(* Logix 5000 AddOnInstructionDefinition export Banner_K50Display_Param_v4; software revision 33.03 *)

TYPE Banner_IOL_Port_v4 :   // UDT that has all of the data items necessary to communicate with a specific Port on a IO-Link Master
STRUCT
   Port_Controlled : INT;   // Each bit represents a port on an IO-Link Master. Set to 1 to tell AOI to control that port.
   Port_Activate : INT;   // Each bit represents a port on an IO-Link Master. When ON that port will process any commands in queue.
   Port_Read : INT;   // Each bit represents a port on an IO-Link Master. Used to determine when device AOI has requested a Read command.
   Port_Write : INT;   // Each bit represents a port on an IO-Link Master. Used to determine when device AOI has requested a Write command.
   Port_RW_Complete : INT;   // Each bit represents a port on an IO-Link Master. Tells device AOI that Read or Write request has been completed.
   Port_Device_Read : INT;
   Data_Transfer : SINT[190];   // Array to transfer data from IO-Master to device AOIs.
END_STRUCT
END_TYPE

TYPE Banner_K50Display_Display_v4 :   // UDT that covers Display Configuration parameters.
STRUCT
   Intensity : SINT;   // 0 = Low, 1 = Medium, 2 = High, 3 = Ultra High
   Orientation : SINT;   // 0 = Standard, 1 = Flipped
   Scroll_Speed : SINT;   // 0 = Off, 1 = Slow, 2 = Medium, 3 = Fast
   Startup_Message : SINT;   // 0 = Off, 1 = Comms Parameter, 2 = Custom
   Startup_String_Delay : DINT;   // 0 to 65535 ms
   Encoding : SINT;   // 0 = ASCII, 1 = Numeric
   Decimal_Type_1 : SINT;   // 0 = Off, 1 = On, 2 = Flash, 3 = Communication, 4 = Power + Communication.
   Decimal_Type_2 : SINT;   // 0 = Off, 1 = On, 2 = Flash, 3 = Communication, 4 = Power + Communication.
   Decimal_Type_3 : SINT;   // 0 = Off, 1 = On, 2 = Flash, 3 = Communication, 4 = Power + Communication.
   Decimal_Type_4 : SINT;   // 0 = Off, 1 = On, 2 = Flash, 3 = Communication, 4 = Power + Communication.
   Startup_String : STRING;
END_STRUCT
END_TYPE

TYPE Banner_K50Display_RD_v4 :   // UDT with all of the Read only parameters for K50 Pro Display.
STRUCT
   Master_Cycle_Time : INT;
   Min_Cycle_Time : INT;
   M_Sequence_Capability : INT;
   IO_Link_Version_ID : INT;
   Process_Data_Input_Length : INT;
   Process_Data_Output_Length : INT;
   Combined_Vendor_ID : DINT;   // IO-Link Vendor ID
   Vendor_ID1 : INT;
   Vendor_ID2 : INT;
   Combined_Device_ID : DINT;   // IO-Link Device ID
   Device_ID1 : INT;
   Device_ID2 : INT;
   Device_ID3 : INT;
   Serial_Number : STRING;
END_STRUCT
END_TYPE

TYPE Banner_K50Display_SP_v4 :   // UDT for K50 Pro Display with the State Parameters structure.
STRUCT
   Type : SINT;   // 0 = Off, 1 = Steady, 2 = Flash, 3 = Two Color Flash, 4 = 50/50, 5 = 50/50 Rotate, 6 = Chase, 7 = Intensity Sweep, 8 = Color Sweep, 9 = Sequence, 10 = Wave, 11 = Double Wave, 12 = Steady Area 1, 13 = Steady Area 2, 14 Alternate Area 1 Area 2
   Direction : SINT;   // 0 = CCW, 1 = CW.
   Pattern : SINT;   // 0 = Flash, 1 = Strobe, 2 = Three Pulse, 3 = SOS, 4 = Random.
   Speed : SINT;   // 0 = Slow, 1 = Medium, 2 = Fast, 3 = Custom.
   Off_Delay_Type : SINT;   // 0 =Leading Edge, 1 = Trailing Edge.
   Off_Delay : DINT;   // 0 to 65535 in ms. Length of time before the device returns to 'touch inactive' state after button is released.
   Static_Sequence : INT;   // 0 to 255. Value describing the LED position of the device.
   Sequence_Start_Location : SINT;   // 0 = LED1, 1 = LED2, 2 = LED3, 3 = LED4, 4 = LED5, 5 = LED6, 6 = LED7, 7 = LED8.
   Color_1 : SINT;   // 0 = Green, 1 = Red, 2 = Orange, 3 = Amber, 4 = Yellow, 5 = Lime Green, 6 = Spring Green, 7 = Cyan, 8 = SKy Blue, 9 = Blue, 10 = Violet, 11 = Magenta, 12 = Rose, 13 = White, 14 Custom 1, 15 = Custom 2.
   Color_1_Intensity : SINT;   // 0 = High, 1 = Medium, 2 = Low, 3 = Off, 4 = Custom.
   Color_2 : SINT;   // 0 = Green, 1 = Red, 2 = Orange, 3 = Amber, 4 = Yellow, 5 = Lime Green, 6 = Spring Green, 7 = Cyan, 8 = SKy Blue, 9 = Blue, 10 = Violet, 11 = Magenta, 12 = Rose, 13 = White, 14 Custom 1, 15 = Custom 2.
   Color_2_Intensity : SINT;   // 0 = High, 1 = Medium, 2 = Low, 3 = Off, 4 = Custom.
END_STRUCT
END_TYPE

TYPE Banner_K50Display_v4 :   // UDT with all of the parameters for K50 Pro Display.
STRUCT
   Initial_Global_Read : BOOL;   // Determines if all of the IO-Link data has been read into the PLC yet
   Command : INT;   // Value placed in here will activate a read or write to a specifc IO-Link Index
   Read : Banner_K50Display_RD_v4;   // All read data
   Write : Banner_K50Display_WD_v4;   // All data that can be written to.
   Archive : Banner_K50Display_WD_v4;   // Archive of the write data.
   Reset : BOOL;
END_STRUCT
END_TYPE

TYPE Banner_K50Display_WD_v4 :   // UDT that stores the Write Data for a K50 Pro Display.
STRUCT
   System_Command : INT;   // See IODD file for list of commands that can be activated via the System Command interface
   Parameter_Access_Lock : SINT;   // Write access to all read/write parameters is block when this bit is ON.
   Data_Storage_Lock : SINT;   // Data storage mechanism is inhibited when bit is ON.
   Local_Parameterization_Lock : SINT;   // Parameteriation via local control elementes is inhibited.
   Local_User_Interface_Lock : SINT;   // Operation of the hmi on the device is disabled.
   Operation_Mode : SINT;   // 0 = Multicolor, 1 = Four State Full Logic, 2 = Advanced, 3 = LED Control, 4 = Demo.
   Custom_Intensity : SINT;   // 0 to 100 %
   Custom_Flash_Rate : INT;   // Range 5 to 200 (.5 to 20 converted rate).
   Restrict_to_Gamut : SINT;   // 0 = Off, 1 = On.
   Touch_Sensitivity : SINT;   // 0 = Low, 1 = Standard, 2 = High.
   Function_1 : SINT;   // 0 = Momentary, 1 = Latched.
   Mute_Enable_1 : SINT;   // 0 = Off, 1 = On.
   Function_2 : SINT;   // 0 = Momentary, 1 = Latched.
   Mute_Enable_2 : SINT;   // 0 = Off, 1 = On.
   On_Delay_1 : DINT;   // 0 to 65535 in ms. Length of time the touch button needs to be pressed to trigger touch active state.
   On_Delay_2 : DINT;   // 0 to 65535 in ms. Length of time the touch button needs to be pressed to trigger touch active state.
   Output_State : SINT;   // 0 = NC, 1 = NO
   Off_Delay_Type_1 : SINT;   // 0 - Leading Edge, 1 = Trailing Edge
   Off_Delay_Type_2 : SINT;   // 0 - Leading Edge, 1 = Trailing Edge
   Off_Delay_1 : DINT;   // Length of time before device returns to touch inactive
   Off_Delay_2 : DINT;   // Length of time before device returns to touch inactive
   State_Parameters : Banner_K50Display_SP_v4[6];   // State Parameters. 1 through 4 will have values.
   CC1_Red : INT;   // 0-255. Custom 1 Red.
   CC1_Green : INT;   // 0-255. Custom 1 Green.
   CC1_Blue : INT;   // 0-255. Custom 1 Blue.
   CC2_Red : INT;   // 0-255. Custom 2 Red.
   CC2_Green : INT;   // 0-255. Custom 2 Green.
   CC2_Blue : INT;   // 0-255. Custom 2 Blue.
   Display_Config : Banner_K50Display_Display_v4;
END_STRUCT
END_TYPE

ADD_ON_INSTRUCTION Banner_K50Display_Param_v4   (* revision 4.2, vendor Banner Engineering *)
// AOI to read and write parameter data to an IO-Link K50 Pro Display.
// Revision note:
// Resolved transfer array index issue.
VAR_IN_OUT
   K50 : Banner_K50Display_v4; {required}
   Port_Data : Banner_IOL_Port_v4; {required}
END_VAR
VAR_INPUT
   Port : DINT; {required}
END_VAR
VAR
   Local_Control : DINT; {access None}
   Global_Read_Command_Value : INT; {access None}
   Global_Write_Command_Value : INT; {access None}
   Command_Being_Processed : BOOL; {access None}
   Update_Archive : BOOL; {access None}
   Index_Write_Control : DINT; {access None}
   Index_Write_Inprocess : INT; {access None}
   Temp_Excess_Gain : DINT[2]; {access None}
   Inprocess_Index : DINT; {access None}
   SP_Index : DINT; {access None}   // State Parameters Index
   SP_Write_Index : DINT; {access None}
   SP_R_Index : DINT; {access None}
   SP_W_Index : DINT; {access None}
END_VAR

ROUTINE Logic   (* ladder *)
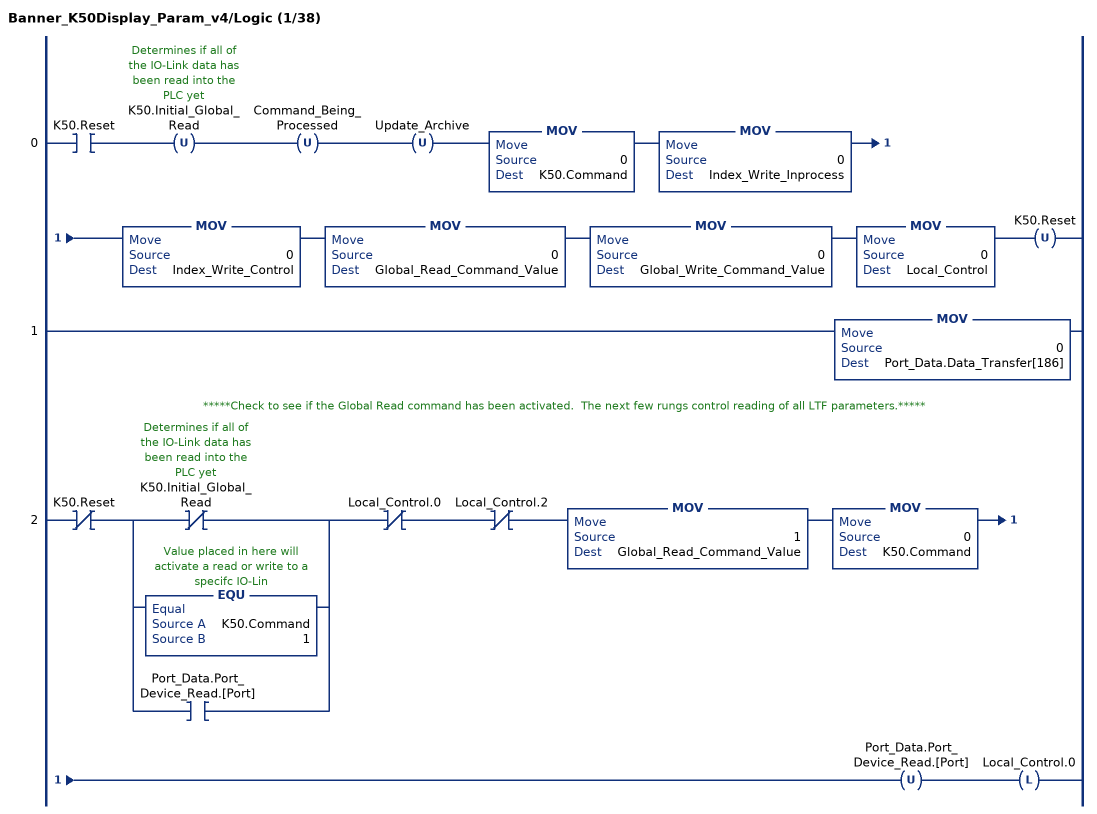
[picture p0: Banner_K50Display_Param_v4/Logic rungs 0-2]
   0: XIC(K50.Reset)OTU(K50.Initial_Global_Read)OTU(Command_Being_Processed)OTU(Update_Archive)MOV(0,K50.Command)MOV(0,Index_Write_Inprocess)MOV(0,Index_Write_Control)MOV(0,Global_Read_Command_Value)MOV(0,Global_Write_Command_Value)MOV(0,Local_Control)OTU(K50.Reset);
   1: MOV(0,Port_Data.Data_Transfer[186]);
   // *****Check to see if the Global Read command has been activated.  The next few rungs control reading of all LTF parameters.*****
   2: XIO(K50.Reset)[XIO(K50.Initial_Global_Read) ,EQU(K50.Command,1) ,XIC(Port_Data.Port_Device_Read.[Port]) ]XIO(Local_Control.0)XIO(Local_Control.2)MOV(1,Global_Read_Command_Value)MOV(0,K50.Command)OTU(Port_Data.Port_Device_Read.[Port])OTL(Local_Control.0);
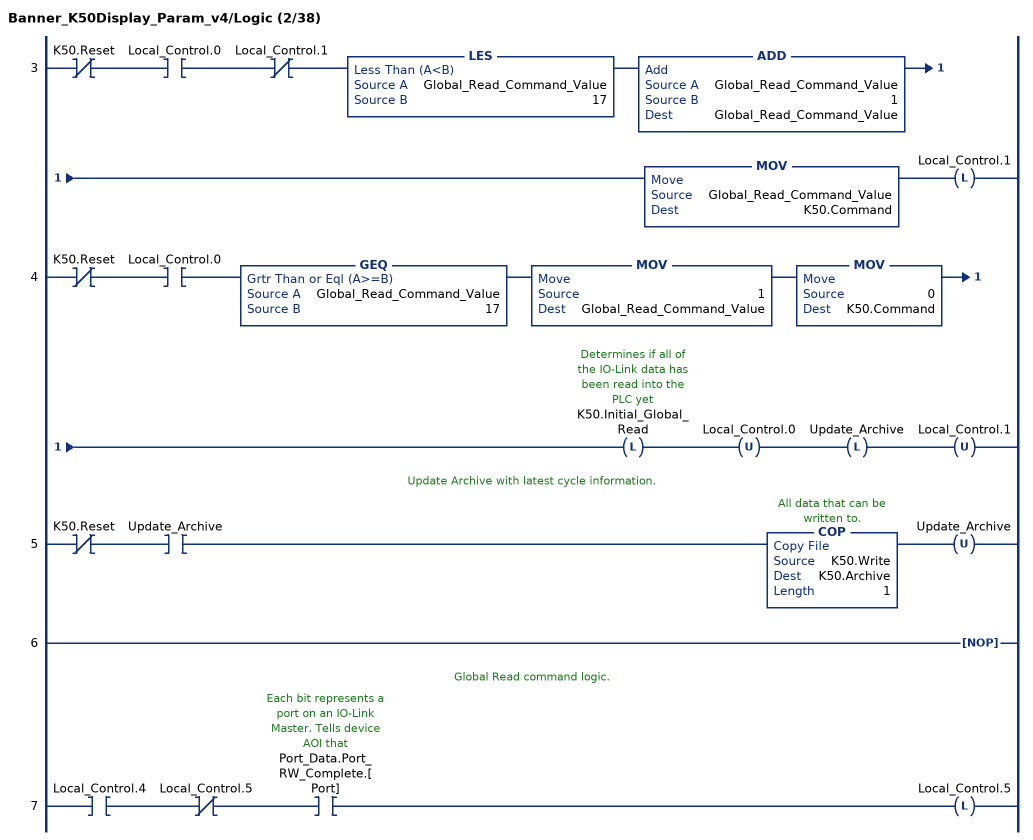
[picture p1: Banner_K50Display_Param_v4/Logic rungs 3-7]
   3: XIO(K50.Reset)XIC(Local_Control.0)XIO(Local_Control.1)LES(Global_Read_Command_Value,17)ADD(Global_Read_Command_Value,1,Global_Read_Command_Value)MOV(Global_Read_Command_Value,K50.Command)OTL(Local_Control.1);
   4: XIO(K50.Reset)XIC(Local_Control.0)GEQ(Global_Read_Command_Value,17)MOV(1,Global_Read_Command_Value)MOV(0,K50.Command)OTL(K50.Initial_Global_Read)OTU(Local_Control.0)OTL(Update_Archive)OTU(Local_Control.1);
   // Update Archive with latest cycle information.
   5: XIO(K50.Reset)XIC(Update_Archive)COP(K50.Write,K50.Archive,1)OTU(Update_Archive);
   6: NOP();
   // Global Read command logic.
   7: XIC(Local_Control.4)XIO(Local_Control.5)XIC(Port_Data.Port_RW_Complete.[Port])OTL(Local_Control.5);
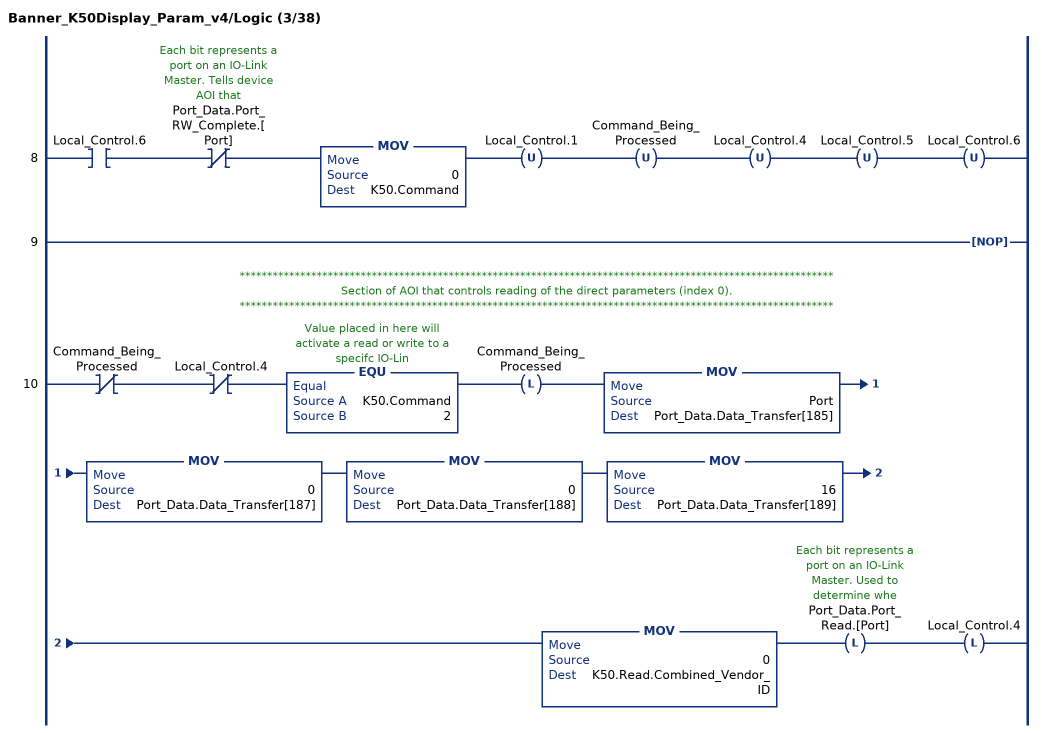
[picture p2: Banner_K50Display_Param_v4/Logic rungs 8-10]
   8: XIC(Local_Control.6)XIO(Port_Data.Port_RW_Complete.[Port])MOV(0,K50.Command)OTU(Local_Control.1)OTU(Command_Being_Processed)OTU(Local_Control.4)OTU(Local_Control.5)OTU(Local_Control.6);
   9: NOP();
   // ************************************************************************************************************
   // Section of AOI that controls reading of the direct parameters (index 0).
   // ************************************************************************************************************
   10: XIO(Command_Being_Processed)XIO(Local_Control.4)EQU(K50.Command,2)OTL(Command_Being_Processed)MOV(Port,Port_Data.Data_Transfer[185])MOV(0,Port_Data.Data_Transfer[187])MOV(0,Port_Data.Data_Transfer[188])MOV(16,Port_Data.Data_Transfer[189])MOV(0,K50.Read.Combined_Vendor_ID)OTL(Port_Data.Port_Read.[Port])OTL(Local_Control.4);
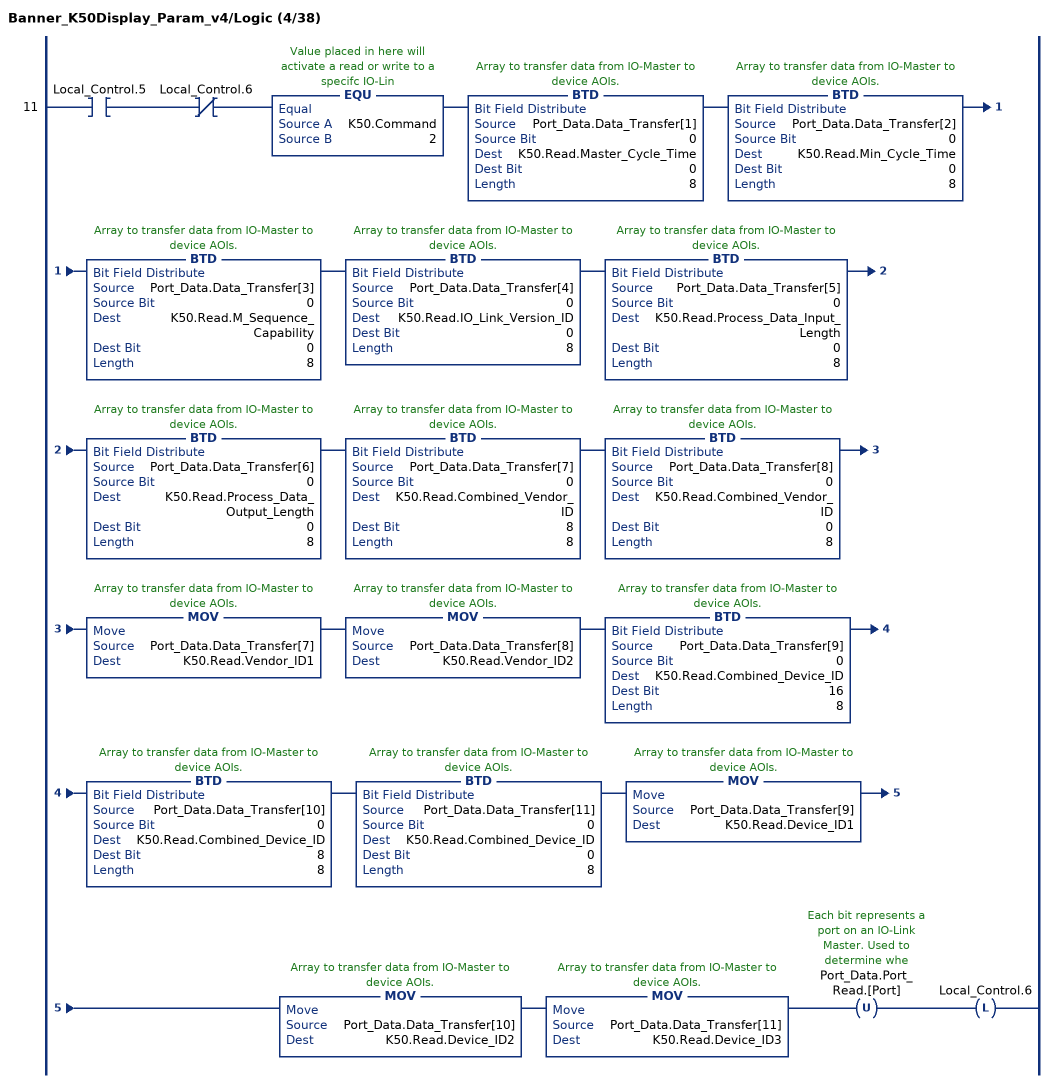
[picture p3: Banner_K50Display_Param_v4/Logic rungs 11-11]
   11: XIC(Local_Control.5)XIO(Local_Control.6)EQU(K50.Command,2)BTD(Port_Data.Data_Transfer[1],0,K50.Read.Master_Cycle_Time,0,8)BTD(Port_Data.Data_Transfer[2],0,K50.Read.Min_Cycle_Time,0,8)BTD(Port_Data.Data_Transfer[3],0,K50.Read.M_Sequence_Capability,0,8)BTD(Port_Data.Data_Transfer[4],0,K50.Read.IO_Link_Version_ID,0,8)BTD(Port_Data.Data_Transfer[5],0,K50.Read.Process_Data_Input_Length,0,8)BTD(Port_Data.Data_Transfer[6],0,K50.Read.Process_Data_Output_Length,0,8)BTD(Port_Data.Data_Transfer[7],0,K50.Read.Combined_Vendor_ID,8,8)BTD(Port_Data.Data_Transfer[8],0,K50.Read.Combined_Vendor_ID,0,8)MOV(Port_Data.Data_Transfer[7],K50.Read.Vendor_ID1)MOV(Port_Data.Data_Transfer[8],K50.Read.Vendor_ID2)BTD(Port_Data.Data_Transfer[9],0,K50.Read.Combined_Device_ID,16,8)BTD(Port_Data.Data_Transfer[10],0,K50.Read.Combined_Device_ID,8,8)BTD(Port_Data.Data_Transfer[11],0,K50.Read.Combined_Device_ID,0,8)MOV(Port_Data.Data_Transfer[9],K50.Read.Device_ID1)MOV(Port_Data.Data_Transfer[10],K50.Read.Device_ID2)MOV(Port_Data.Data_Transfer[11],K50.Read.Device_ID3)OTU(Port_Data.Port_Read.[Port])OTL(Local_Control.6);
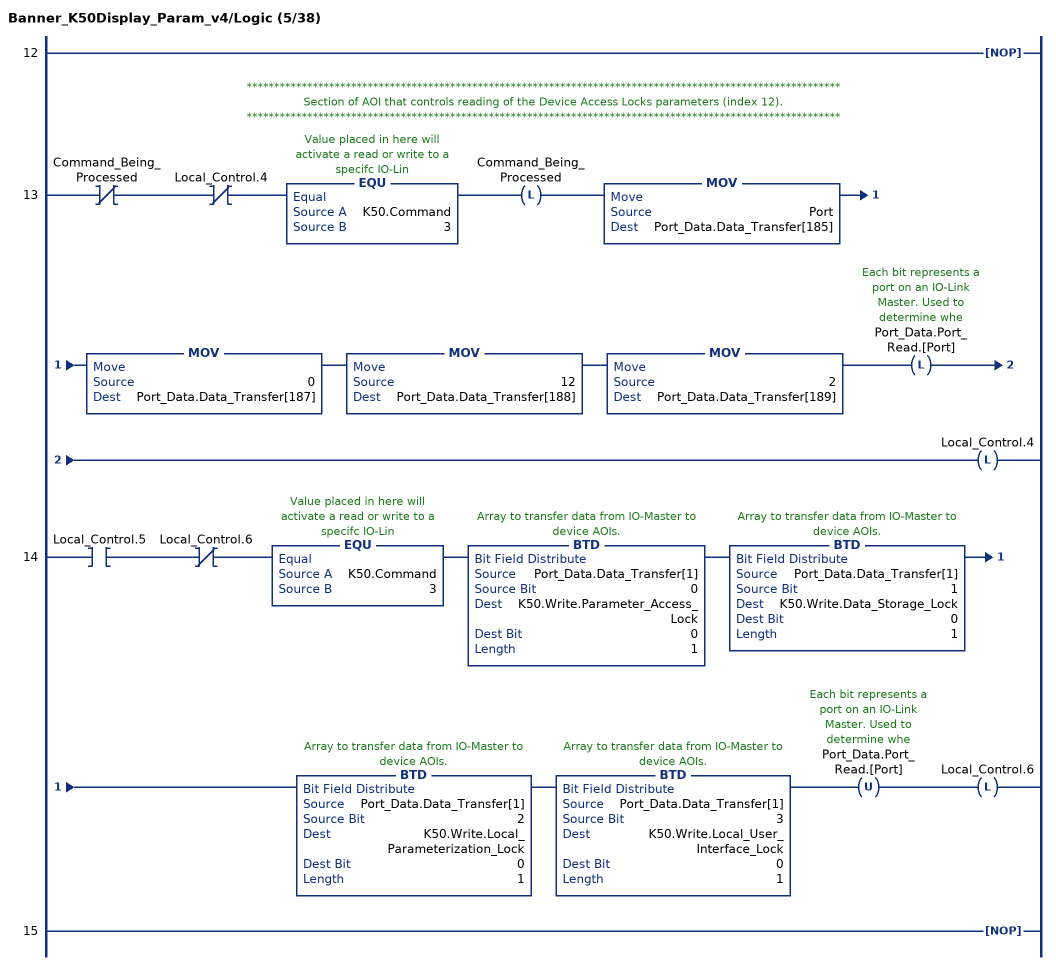
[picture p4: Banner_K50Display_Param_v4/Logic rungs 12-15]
   12: NOP();
   // ************************************************************************************************************
   // Section of AOI that controls reading of the Device Access Locks parameters (index 12).
   // ************************************************************************************************************
   13: XIO(Command_Being_Processed)XIO(Local_Control.4)EQU(K50.Command,3)OTL(Command_Being_Processed)MOV(Port,Port_Data.Data_Transfer[185])MOV(0,Port_Data.Data_Transfer[187])MOV(12,Port_Data.Data_Transfer[188])MOV(2,Port_Data.Data_Transfer[189])OTL(Port_Data.Port_Read.[Port])OTL(Local_Control.4);
   14: XIC(Local_Control.5)XIO(Local_Control.6)EQU(K50.Command,3)BTD(Port_Data.Data_Transfer[1],0,K50.Write.Parameter_Access_Lock,0,1)BTD(Port_Data.Data_Transfer[1],1,K50.Write.Data_Storage_Lock,0,1)BTD(Port_Data.Data_Transfer[1],2,K50.Write.Local_Parameterization_Lock,0,1)BTD(Port_Data.Data_Transfer[1],3,K50.Write.Local_User_Interface_Lock,0,1)OTU(Port_Data.Port_Read.[Port])OTL(Local_Control.6);
   15: NOP();
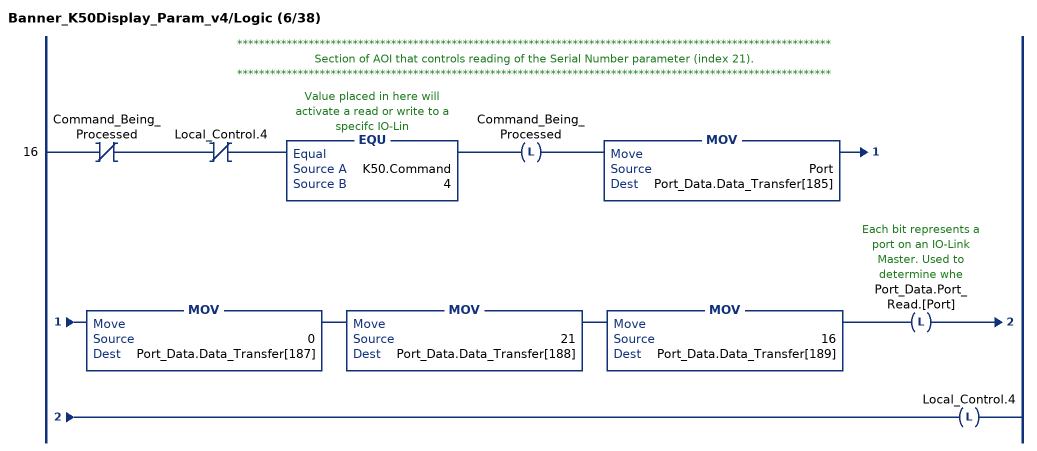
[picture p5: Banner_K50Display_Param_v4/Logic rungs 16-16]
   // ************************************************************************************************************
   // Section of AOI that controls reading of the Serial Number parameter (index 21).
   // ************************************************************************************************************
   16: XIO(Command_Being_Processed)XIO(Local_Control.4)EQU(K50.Command,4)OTL(Command_Being_Processed)MOV(Port,Port_Data.Data_Transfer[185])MOV(0,Port_Data.Data_Transfer[187])MOV(21,Port_Data.Data_Transfer[188])MOV(16,Port_Data.Data_Transfer[189])OTL(Port_Data.Port_Read.[Port])OTL(Local_Control.4);
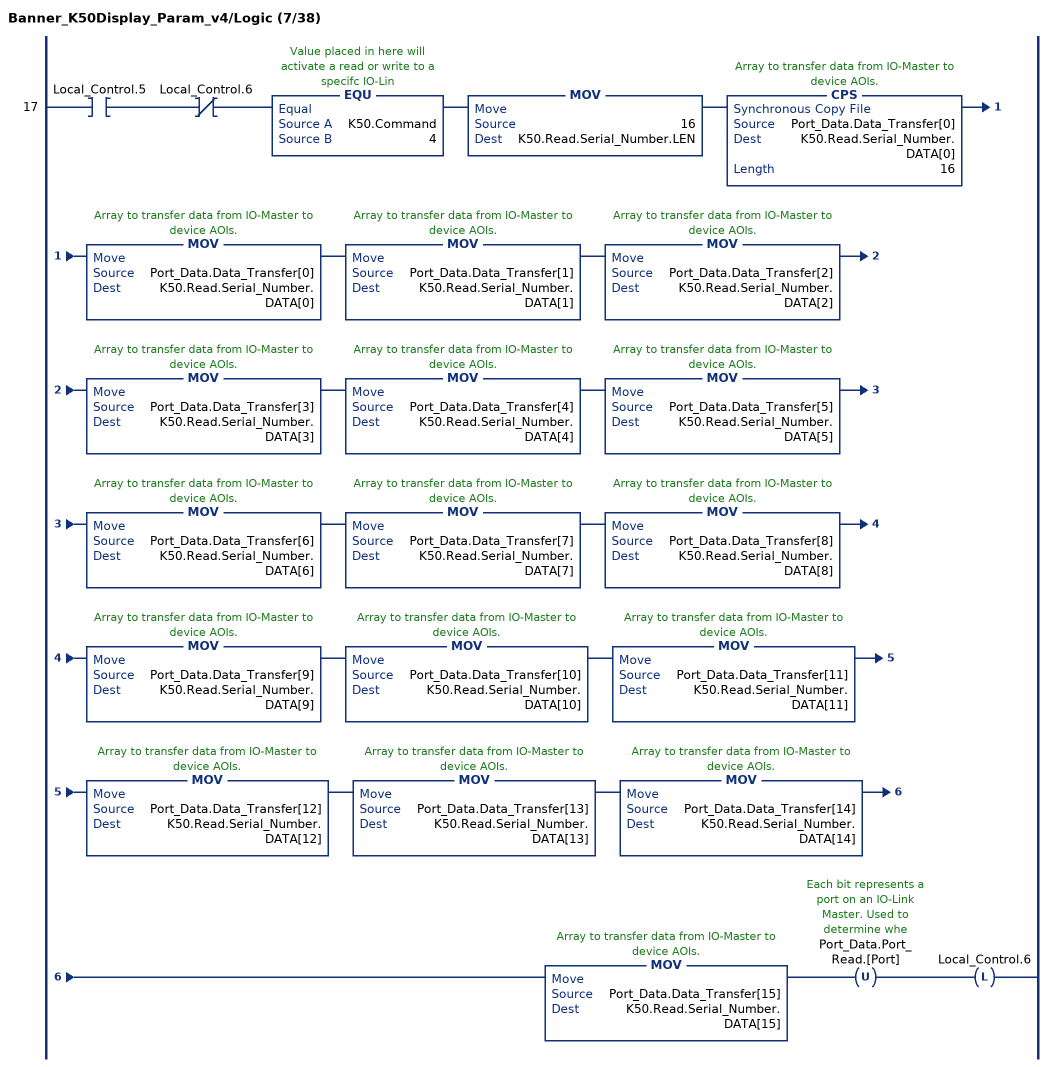
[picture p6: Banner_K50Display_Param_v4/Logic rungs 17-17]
   17: XIC(Local_Control.5)XIO(Local_Control.6)EQU(K50.Command,4)MOV(16,K50.Read.Serial_Number.LEN)CPS(Port_Data.Data_Transfer[0],K50.Read.Serial_Number.DATA[0],16)MOV(Port_Data.Data_Transfer[0],K50.Read.Serial_Number.DATA[0])MOV(Port_Data.Data_Transfer[1],K50.Read.Serial_Number.DATA[1])MOV(Port_Data.Data_Transfer[2],K50.Read.Serial_Number.DATA[2])MOV(Port_Data.Data_Transfer[3],K50.Read.Serial_Number.DATA[3])MOV(Port_Data.Data_Transfer[4],K50.Read.Serial_Number.DATA[4])MOV(Port_Data.Data_Transfer[5],K50.Read.Serial_Number.DATA[5])MOV(Port_Data.Data_Transfer[6],K50.Read.Serial_Number.DATA[6])MOV(Port_Data.Data_Transfer[7],K50.Read.Serial_Number.DATA[7])MOV(Port_Data.Data_Transfer[8],K50.Read.Serial_Number.DATA[8])MOV(Port_Data.Data_Transfer[9],K50.Read.Serial_Number.DATA[9])MOV(Port_Data.Data_Transfer[10],K50.Read.Serial_Number.DATA[10])MOV(Port_Data.Data_Transfer[11],K50.Read.Serial_Number.DATA[11])MOV(Port_Data.Data_Transfer[12],K50.Read.Serial_Number.DATA[12])MOV(Port_Data.Data_Transfer[13],K50.Read.Serial_Number.DATA[13])MOV(Port_Data.Data_Transfer[14],K50.Read.Serial_Number.DATA[14])MOV(Port_Data.Data_Transfer[15],K50.Read.Serial_Number.DATA[15])OTU(Port_Data.Port_Read.[Port])OTL(Local_Control.6);
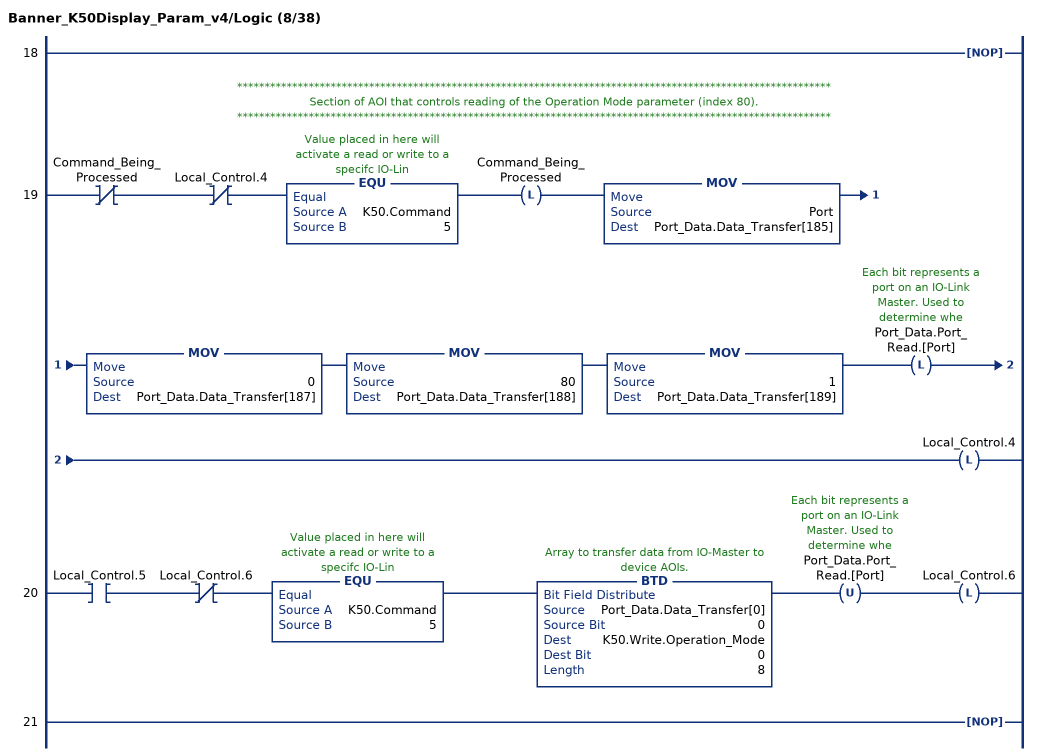
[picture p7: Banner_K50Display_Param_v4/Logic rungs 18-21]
   18: NOP();
   // ************************************************************************************************************
   // Section of AOI that controls reading of the Operation Mode parameter (index 80).
   // ************************************************************************************************************
   19: XIO(Command_Being_Processed)XIO(Local_Control.4)EQU(K50.Command,5)OTL(Command_Being_Processed)MOV(Port,Port_Data.Data_Transfer[185])MOV(0,Port_Data.Data_Transfer[187])MOV(80,Port_Data.Data_Transfer[188])MOV(1,Port_Data.Data_Transfer[189])OTL(Port_Data.Port_Read.[Port])OTL(Local_Control.4);
   20: XIC(Local_Control.5)XIO(Local_Control.6)EQU(K50.Command,5)BTD(Port_Data.Data_Transfer[0],0,K50.Write.Operation_Mode,0,8)OTU(Port_Data.Port_Read.[Port])OTL(Local_Control.6);
   21: NOP();
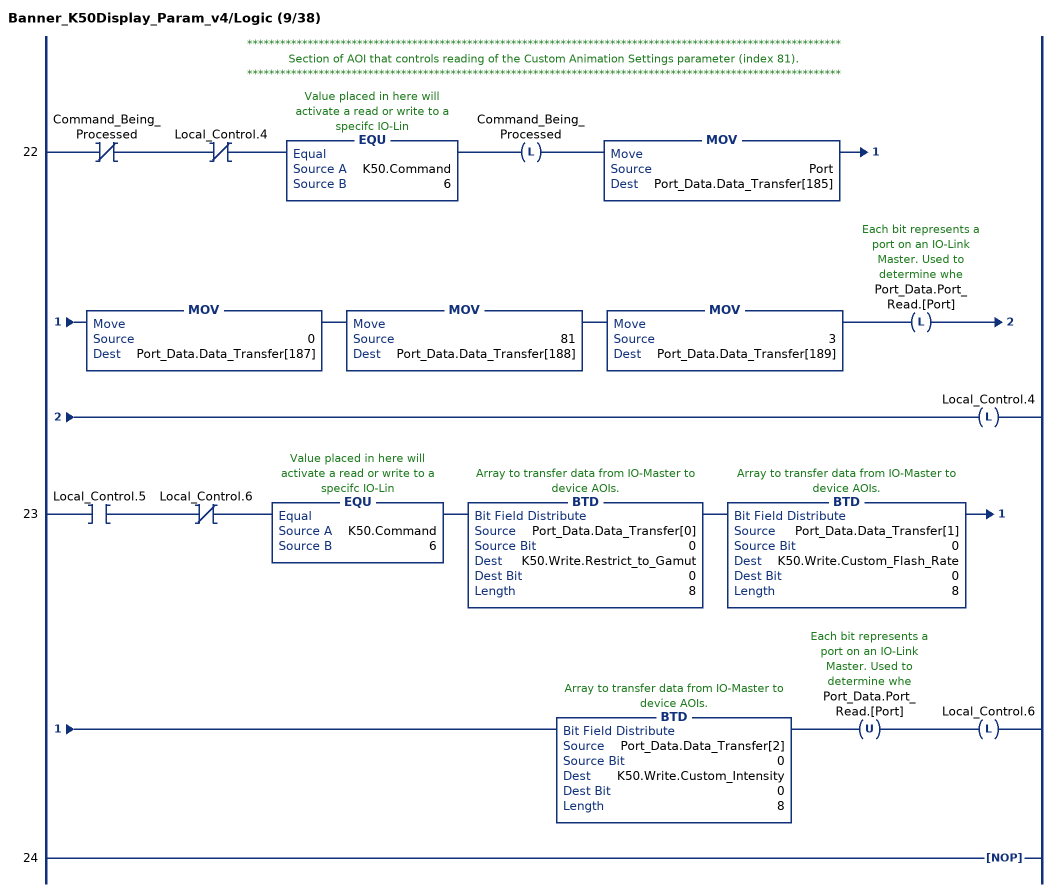
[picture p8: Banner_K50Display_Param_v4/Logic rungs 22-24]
   // ************************************************************************************************************
   // Section of AOI that controls reading of the Custom Animation Settings parameter (index 81).
   // ************************************************************************************************************
   22: XIO(Command_Being_Processed)XIO(Local_Control.4)EQU(K50.Command,6)OTL(Command_Being_Processed)MOV(Port,Port_Data.Data_Transfer[185])MOV(0,Port_Data.Data_Transfer[187])MOV(81,Port_Data.Data_Transfer[188])MOV(3,Port_Data.Data_Transfer[189])OTL(Port_Data.Port_Read.[Port])OTL(Local_Control.4);
   23: XIC(Local_Control.5)XIO(Local_Control.6)EQU(K50.Command,6)BTD(Port_Data.Data_Transfer[0],0,K50.Write.Restrict_to_Gamut,0,8)BTD(Port_Data.Data_Transfer[1],0,K50.Write.Custom_Flash_Rate,0,8)BTD(Port_Data.Data_Transfer[2],0,K50.Write.Custom_Intensity,0,8)OTU(Port_Data.Port_Read.[Port])OTL(Local_Control.6);
   24: NOP();
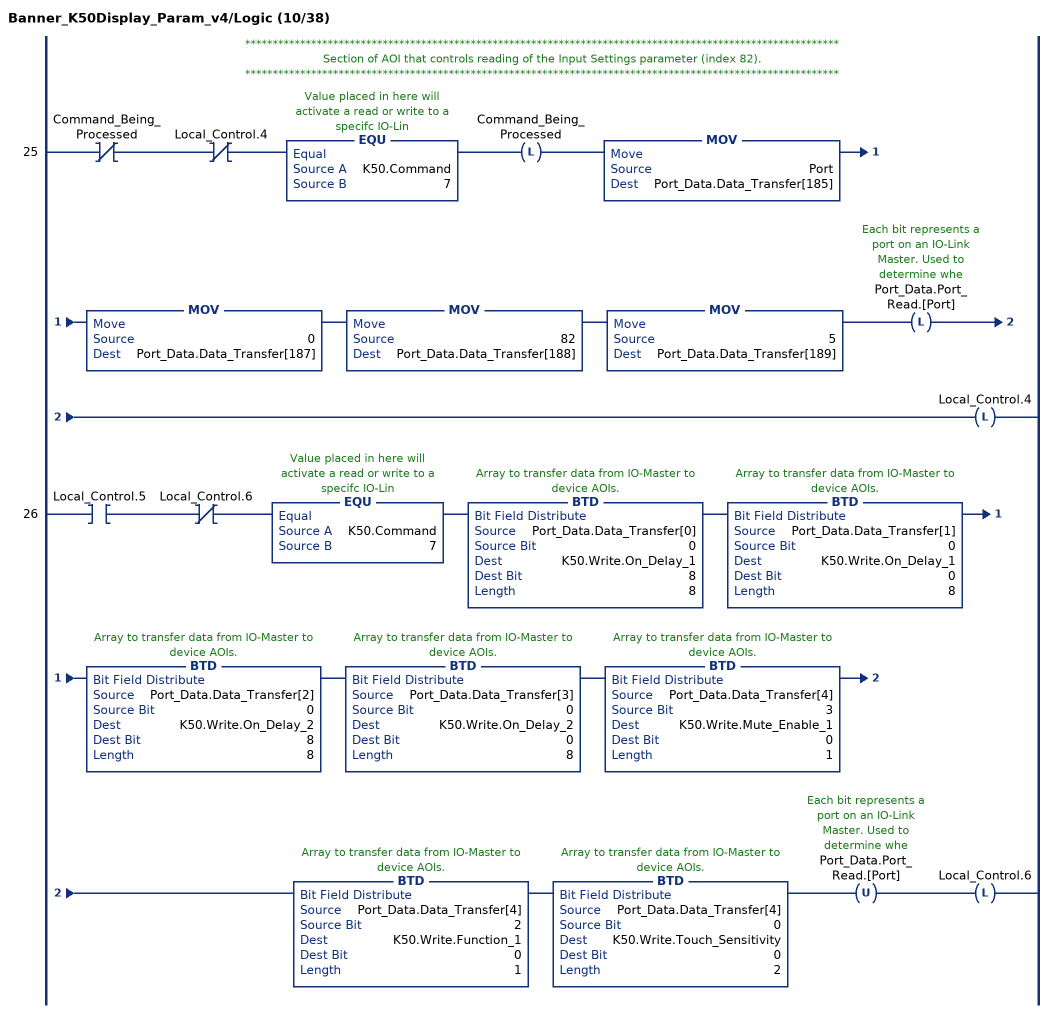
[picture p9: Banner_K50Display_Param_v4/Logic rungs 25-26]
   // ************************************************************************************************************
   // Section of AOI that controls reading of the Input Settings parameter (index 82).
   // ************************************************************************************************************
   25: XIO(Command_Being_Processed)XIO(Local_Control.4)EQU(K50.Command,7)OTL(Command_Being_Processed)MOV(Port,Port_Data.Data_Transfer[185])MOV(0,Port_Data.Data_Transfer[187])MOV(82,Port_Data.Data_Transfer[188])MOV(5,Port_Data.Data_Transfer[189])OTL(Port_Data.Port_Read.[Port])OTL(Local_Control.4);
   26: XIC(Local_Control.5)XIO(Local_Control.6)EQU(K50.Command,7)BTD(Port_Data.Data_Transfer[0],0,K50.Write.On_Delay_1,8,8)BTD(Port_Data.Data_Transfer[1],0,K50.Write.On_Delay_1,0,8)BTD(Port_Data.Data_Transfer[2],0,K50.Write.On_Delay_2,8,8)BTD(Port_Data.Data_Transfer[3],0,K50.Write.On_Delay_2,0,8)BTD(Port_Data.Data_Transfer[4],3,K50.Write.Mute_Enable_1,0,1)BTD(Port_Data.Data_Transfer[4],2,K50.Write.Function_1,0,1)BTD(Port_Data.Data_Transfer[4],0,K50.Write.Touch_Sensitivity,0,2)OTU(Port_Data.Port_Read.[Port])OTL(Local_Control.6);
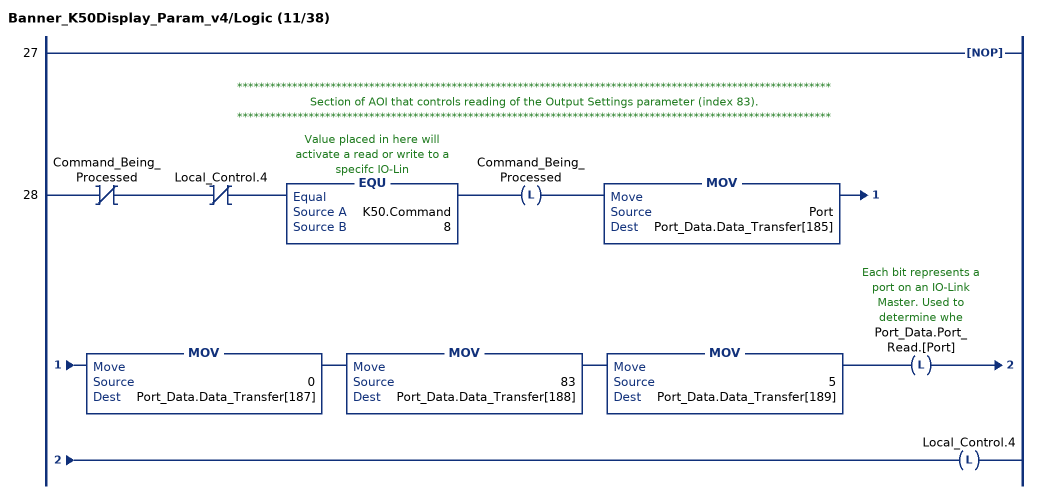
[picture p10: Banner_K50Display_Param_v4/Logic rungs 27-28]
   27: NOP();
   // ************************************************************************************************************
   // Section of AOI that controls reading of the Output Settings parameter (index 83).
   // ************************************************************************************************************
   28: XIO(Command_Being_Processed)XIO(Local_Control.4)EQU(K50.Command,8)OTL(Command_Being_Processed)MOV(Port,Port_Data.Data_Transfer[185])MOV(0,Port_Data.Data_Transfer[187])MOV(83,Port_Data.Data_Transfer[188])MOV(5,Port_Data.Data_Transfer[189])OTL(Port_Data.Port_Read.[Port])OTL(Local_Control.4);
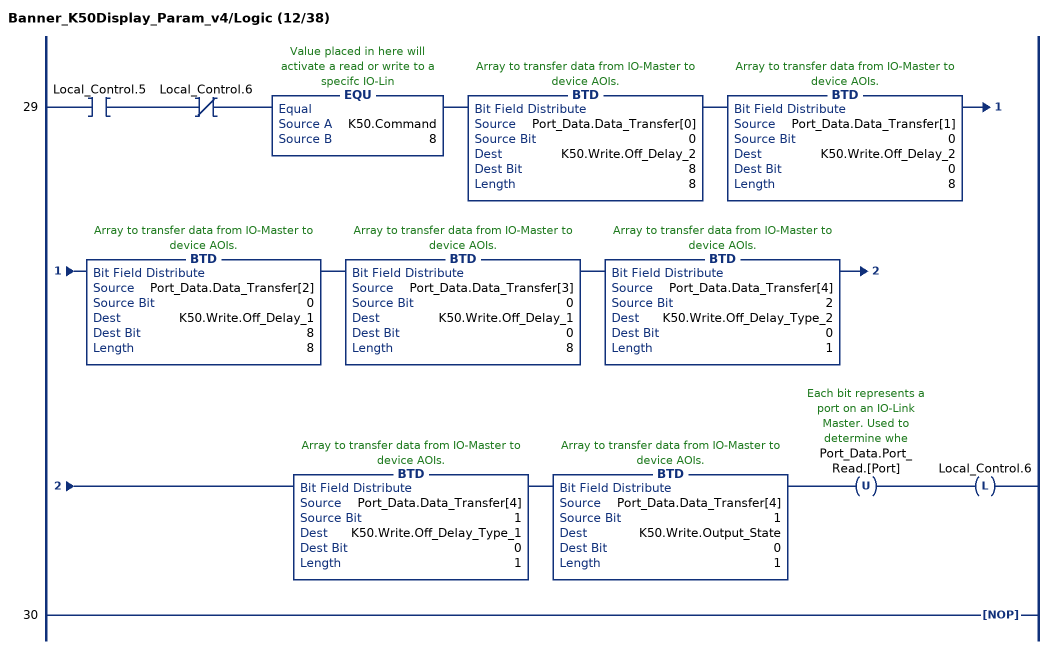
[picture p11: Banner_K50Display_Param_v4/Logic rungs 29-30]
   29: XIC(Local_Control.5)XIO(Local_Control.6)EQU(K50.Command,8)BTD(Port_Data.Data_Transfer[0],0,K50.Write.Off_Delay_2,8,8)BTD(Port_Data.Data_Transfer[1],0,K50.Write.Off_Delay_2,0,8)BTD(Port_Data.Data_Transfer[2],0,K50.Write.Off_Delay_1,8,8)BTD(Port_Data.Data_Transfer[3],0,K50.Write.Off_Delay_1,0,8)BTD(Port_Data.Data_Transfer[4],2,K50.Write.Off_Delay_Type_2,0,1)BTD(Port_Data.Data_Transfer[4],1,K50.Write.Off_Delay_Type_1,0,1)BTD(Port_Data.Data_Transfer[4],1,K50.Write.Output_State,0,1)OTU(Port_Data.Port_Read.[Port])OTL(Local_Control.6);
   30: NOP();
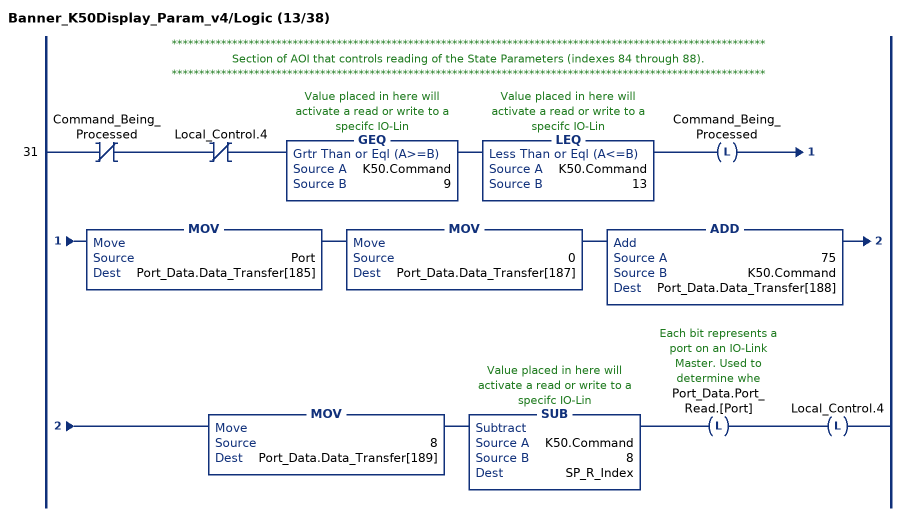
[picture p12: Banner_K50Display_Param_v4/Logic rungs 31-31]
   // ************************************************************************************************************
   // Section of AOI that controls reading of the State Parameters (indexes 84 through 88).
   // ************************************************************************************************************
   31: XIO(Command_Being_Processed)XIO(Local_Control.4)GEQ(K50.Command,9)LEQ(K50.Command,13)OTL(Command_Being_Processed)MOV(Port,Port_Data.Data_Transfer[185])MOV(0,Port_Data.Data_Transfer[187])ADD(75,K50.Command,Port_Data.Data_Transfer[188])MOV(8,Port_Data.Data_Transfer[189])SUB(K50.Command,8,SP_R_Index)OTL(Port_Data.Port_Read.[Port])OTL(Local_Control.4);
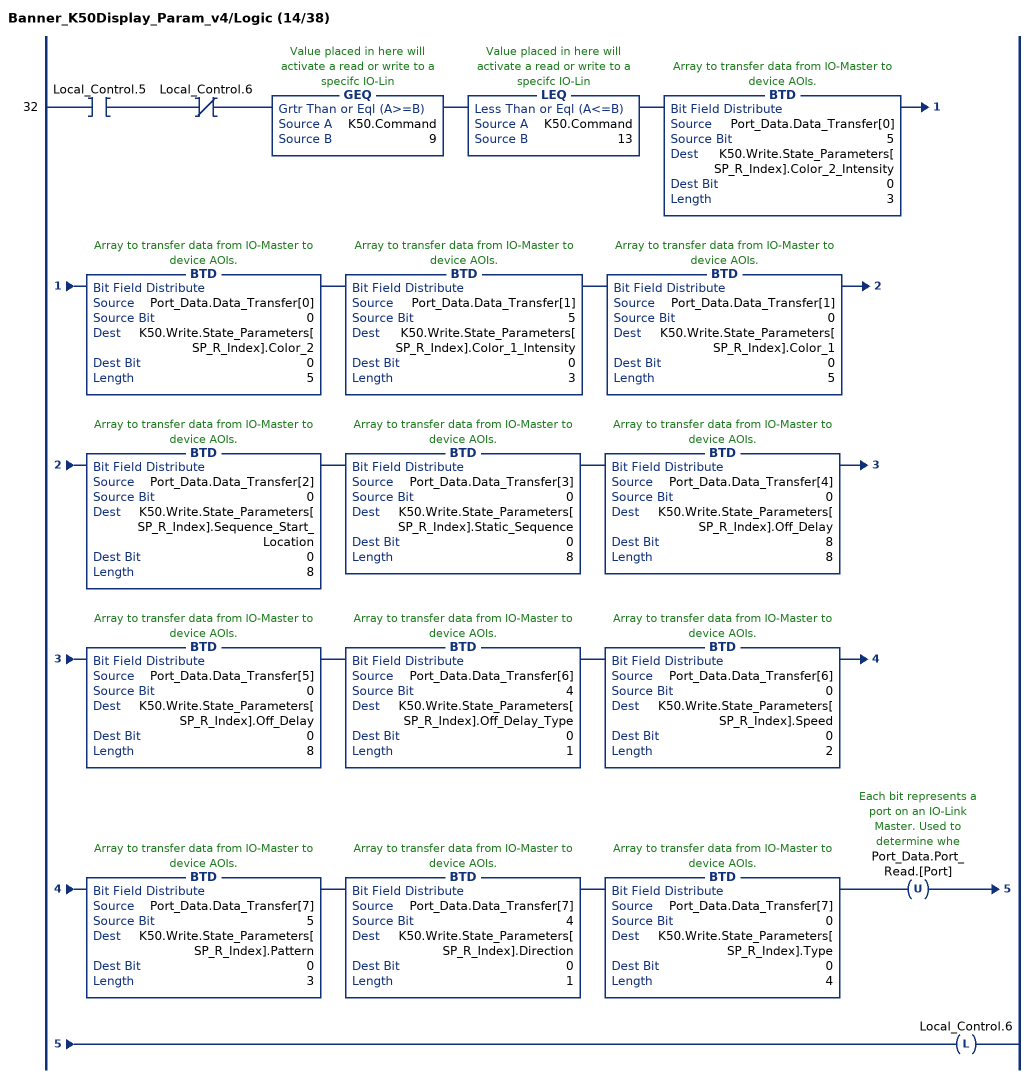
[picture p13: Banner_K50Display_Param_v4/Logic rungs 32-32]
   32: XIC(Local_Control.5)XIO(Local_Control.6)GEQ(K50.Command,9)LEQ(K50.Command,13)BTD(Port_Data.Data_Transfer[0],5,K50.Write.State_Parameters[SP_R_Index].Color_2_Intensity,0,3)BTD(Port_Data.Data_Transfer[0],0,K50.Write.State_Parameters[SP_R_Index].Color_2,0,5)BTD(Port_Data.Data_Transfer[1],5,K50.Write.State_Parameters[SP_R_Index].Color_1_Intensity,0,3)BTD(Port_Data.Data_Transfer[1],0,K50.Write.State_Parameters[SP_R_Index].Color_1,0,5)BTD(Port_Data.Data_Transfer[2],0,K50.Write.State_Parameters[SP_R_Index].Sequence_Start_Location,0,8)BTD(Port_Data.Data_Transfer[3],0,K50.Write.State_Parameters[SP_R_Index].Static_Sequence,0,8)BTD(Port_Data.Data_Transfer[4],0,K50.Write.State_Parameters[SP_R_Index].Off_Delay,8,8)BTD(Port_Data.Data_Transfer[5],0,K50.Write.State_Parameters[SP_R_Index].Off_Delay,0,8)BTD(Port_Data.Data_Transfer[6],4,K50.Write.State_Parameters[SP_R_Index].Off_Delay_Type,0,1)BTD(Port_Data.Data_Transfer[6],0,K50.Write.State_Parameters[SP_R_Index].Speed,0,2)BTD(Port_Data.Data_Transfer[7],5,K50.Write.State_Parameters[SP_R_Index].Pattern,0,3)BTD(Port_Data.Data_Transfer[7],4,K50.Write.State_Parameters[SP_R_Index].Direction,0,1)BTD(Port_Data.Data_Transfer[7],0,K50.Write.State_Parameters[SP_R_Index].Type,0,4)OTU(Port_Data.Port_Read.[Port])OTL(Local_Control.6);
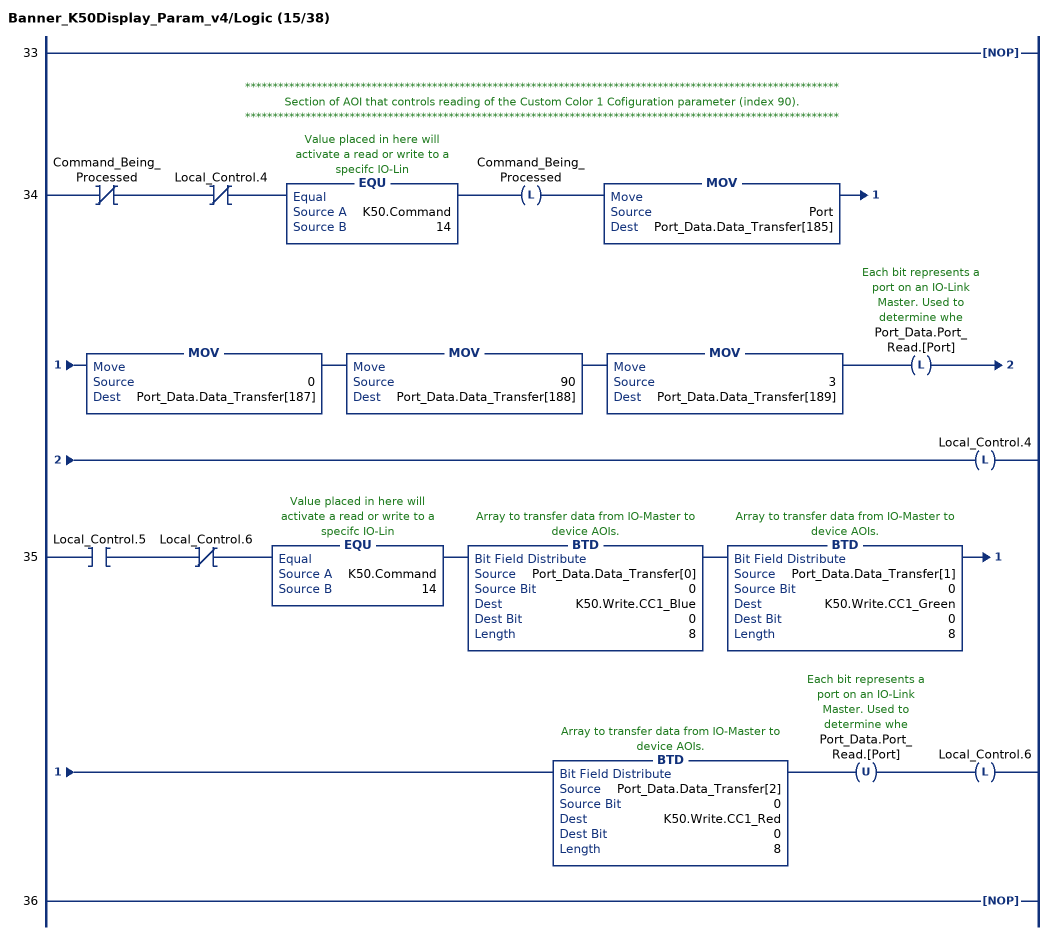
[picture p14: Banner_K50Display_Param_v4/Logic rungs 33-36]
   33: NOP();
   // ************************************************************************************************************
   // Section of AOI that controls reading of the Custom Color 1 Cofiguration parameter (index 90).
   // ************************************************************************************************************
   34: XIO(Command_Being_Processed)XIO(Local_Control.4)EQU(K50.Command,14)OTL(Command_Being_Processed)MOV(Port,Port_Data.Data_Transfer[185])MOV(0,Port_Data.Data_Transfer[187])MOV(90,Port_Data.Data_Transfer[188])MOV(3,Port_Data.Data_Transfer[189])OTL(Port_Data.Port_Read.[Port])OTL(Local_Control.4);
   35: XIC(Local_Control.5)XIO(Local_Control.6)EQU(K50.Command,14)BTD(Port_Data.Data_Transfer[0],0,K50.Write.CC1_Blue,0,8)BTD(Port_Data.Data_Transfer[1],0,K50.Write.CC1_Green,0,8)BTD(Port_Data.Data_Transfer[2],0,K50.Write.CC1_Red,0,8)OTU(Port_Data.Port_Read.[Port])OTL(Local_Control.6);
   36: NOP();
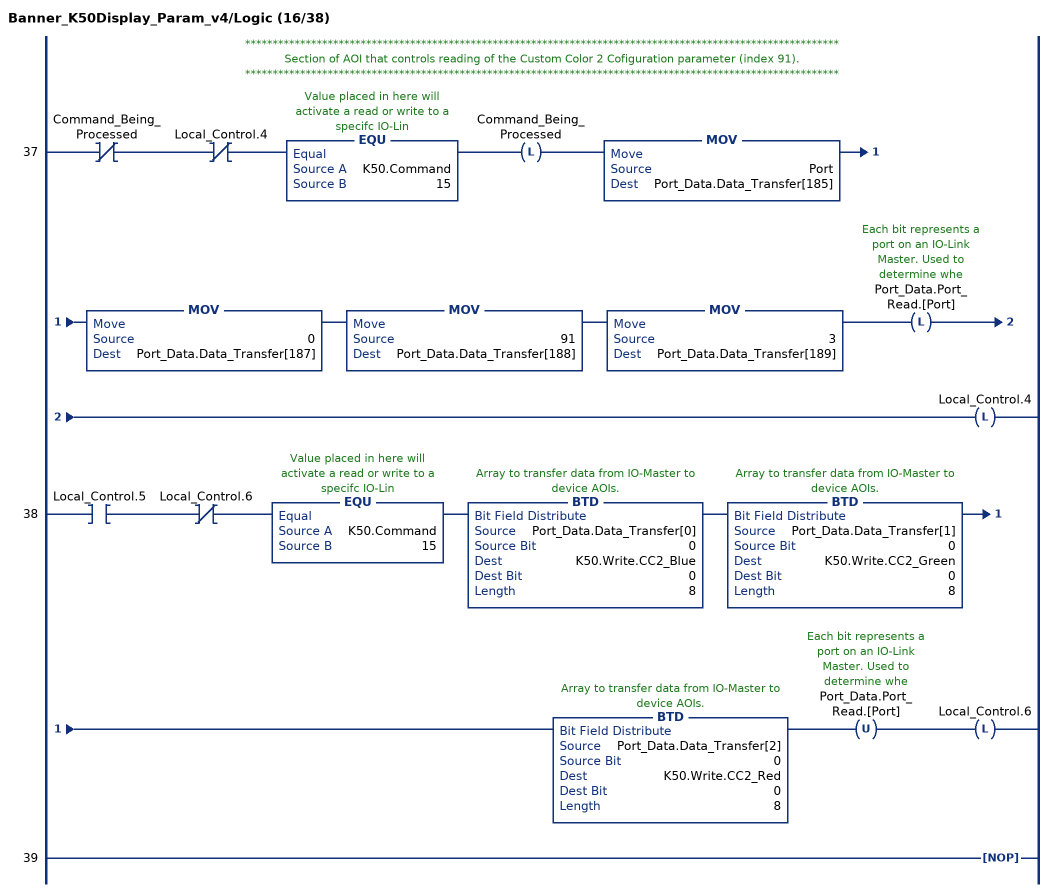
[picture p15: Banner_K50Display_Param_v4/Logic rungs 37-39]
   // ************************************************************************************************************
   // Section of AOI that controls reading of the Custom Color 2 Cofiguration parameter (index 91).
   // ************************************************************************************************************
   37: XIO(Command_Being_Processed)XIO(Local_Control.4)EQU(K50.Command,15)OTL(Command_Being_Processed)MOV(Port,Port_Data.Data_Transfer[185])MOV(0,Port_Data.Data_Transfer[187])MOV(91,Port_Data.Data_Transfer[188])MOV(3,Port_Data.Data_Transfer[189])OTL(Port_Data.Port_Read.[Port])OTL(Local_Control.4);
   38: XIC(Local_Control.5)XIO(Local_Control.6)EQU(K50.Command,15)BTD(Port_Data.Data_Transfer[0],0,K50.Write.CC2_Blue,0,8)BTD(Port_Data.Data_Transfer[1],0,K50.Write.CC2_Green,0,8)BTD(Port_Data.Data_Transfer[2],0,K50.Write.CC2_Red,0,8)OTU(Port_Data.Port_Read.[Port])OTL(Local_Control.6);
   39: NOP();
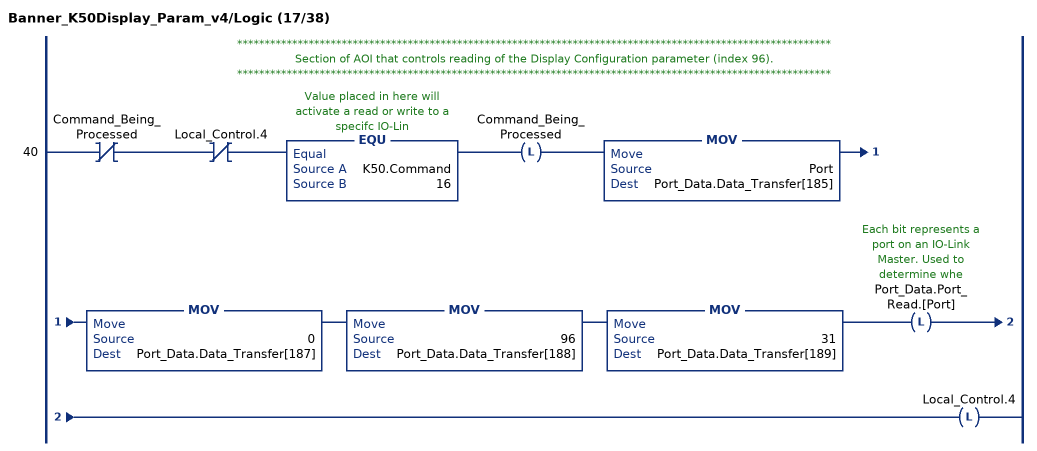
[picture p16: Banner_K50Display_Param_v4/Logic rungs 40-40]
   // ************************************************************************************************************
   // Section of AOI that controls reading of the Display Configuration parameter (index 96).
   // ************************************************************************************************************
   40: XIO(Command_Being_Processed)XIO(Local_Control.4)EQU(K50.Command,16)OTL(Command_Being_Processed)MOV(Port,Port_Data.Data_Transfer[185])MOV(0,Port_Data.Data_Transfer[187])MOV(96,Port_Data.Data_Transfer[188])MOV(31,Port_Data.Data_Transfer[189])OTL(Port_Data.Port_Read.[Port])OTL(Local_Control.4);
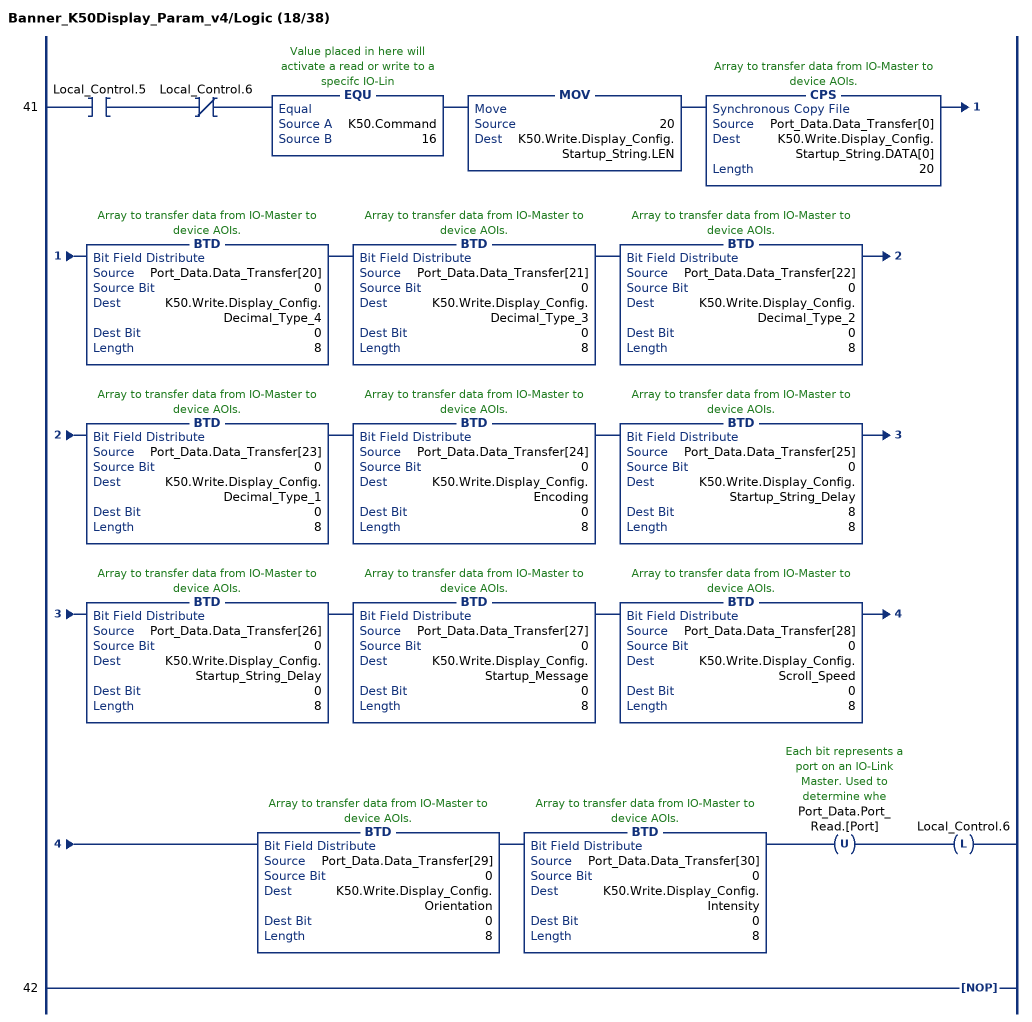
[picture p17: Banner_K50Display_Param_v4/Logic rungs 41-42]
   41: XIC(Local_Control.5)XIO(Local_Control.6)EQU(K50.Command,16)MOV(20,K50.Write.Display_Config.Startup_String.LEN)CPS(Port_Data.Data_Transfer[0],K50.Write.Display_Config.Startup_String.DATA[0],20)BTD(Port_Data.Data_Transfer[20],0,K50.Write.Display_Config.Decimal_Type_4,0,8)BTD(Port_Data.Data_Transfer[21],0,K50.Write.Display_Config.Decimal_Type_3,0,8)BTD(Port_Data.Data_Transfer[22],0,K50.Write.Display_Config.Decimal_Type_2,0,8)BTD(Port_Data.Data_Transfer[23],0,K50.Write.Display_Config.Decimal_Type_1,0,8)BTD(Port_Data.Data_Transfer[24],0,K50.Write.Display_Config.Encoding,0,8)BTD(Port_Data.Data_Transfer[25],0,K50.Write.Display_Config.Startup_String_Delay,8,8)BTD(Port_Data.Data_Transfer[26],0,K50.Write.Display_Config.Startup_String_Delay,0,8)BTD(Port_Data.Data_Transfer[27],0,K50.Write.Display_Config.Startup_Message,0,8)BTD(Port_Data.Data_Transfer[28],0,K50.Write.Display_Config.Scroll_Speed,0,8)BTD(Port_Data.Data_Transfer[29],0,K50.Write.Display_Config.Orientation,0,8)BTD(Port_Data.Data_Transfer[30],0,K50.Write.Display_Config.Intensity,0,8)OTU(Port_Data.Port_Read.[Port])OTL(Local_Control.6);
   42: NOP();
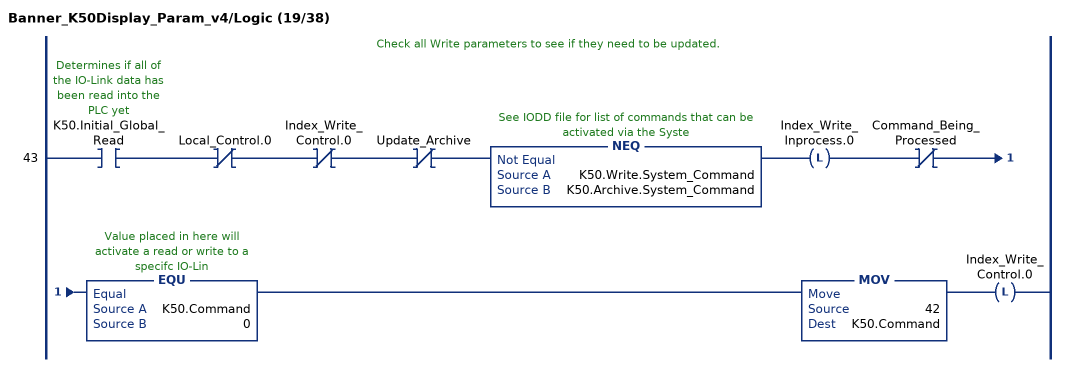
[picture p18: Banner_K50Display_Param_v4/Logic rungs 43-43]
   // Check all Write parameters to see if they need to be updated.
   43: XIC(K50.Initial_Global_Read)XIO(Local_Control.0)XIO(Index_Write_Control.0)XIO(Update_Archive)NEQ(K50.Write.System_Command,K50.Archive.System_Command)OTL(Index_Write_Inprocess.0)XIO(Command_Being_Processed)EQU(K50.Command,0)MOV(42,K50.Command)OTL(Index_Write_Control.0);
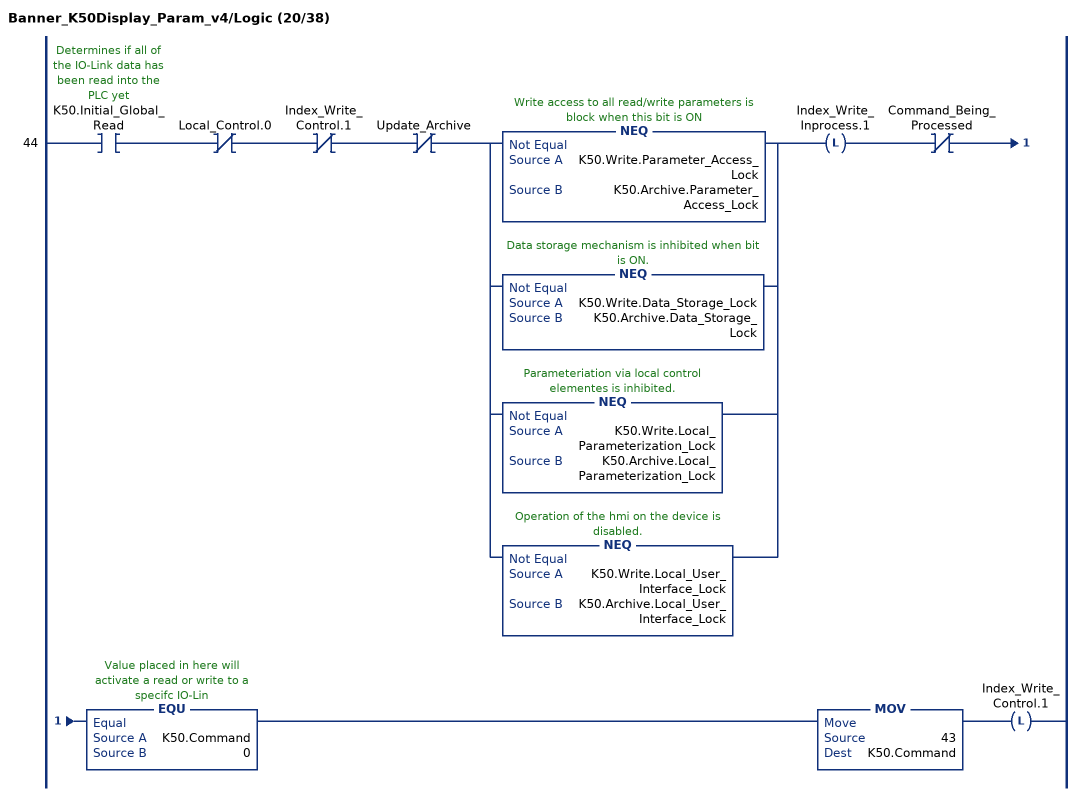
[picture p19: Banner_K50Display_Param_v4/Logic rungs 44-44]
   44: XIC(K50.Initial_Global_Read)XIO(Local_Control.0)XIO(Index_Write_Control.1)XIO(Update_Archive)[NEQ(K50.Write.Parameter_Access_Lock,K50.Archive.Parameter_Access_Lock) ,NEQ(K50.Write.Data_Storage_Lock,K50.Archive.Data_Storage_Lock) ,NEQ(K50.Write.Local_Parameterization_Lock,K50.Archive.Local_Parameterization_Lock) ,NEQ(K50.Write.Local_User_Interface_Lock,K50.Archive.Local_User_Interface_Lock) ]OTL(Index_Write_Inprocess.1)XIO(Command_Being_Processed)EQU(K50.Command,0)MOV(43,K50.Command)OTL(Index_Write_Control.1);
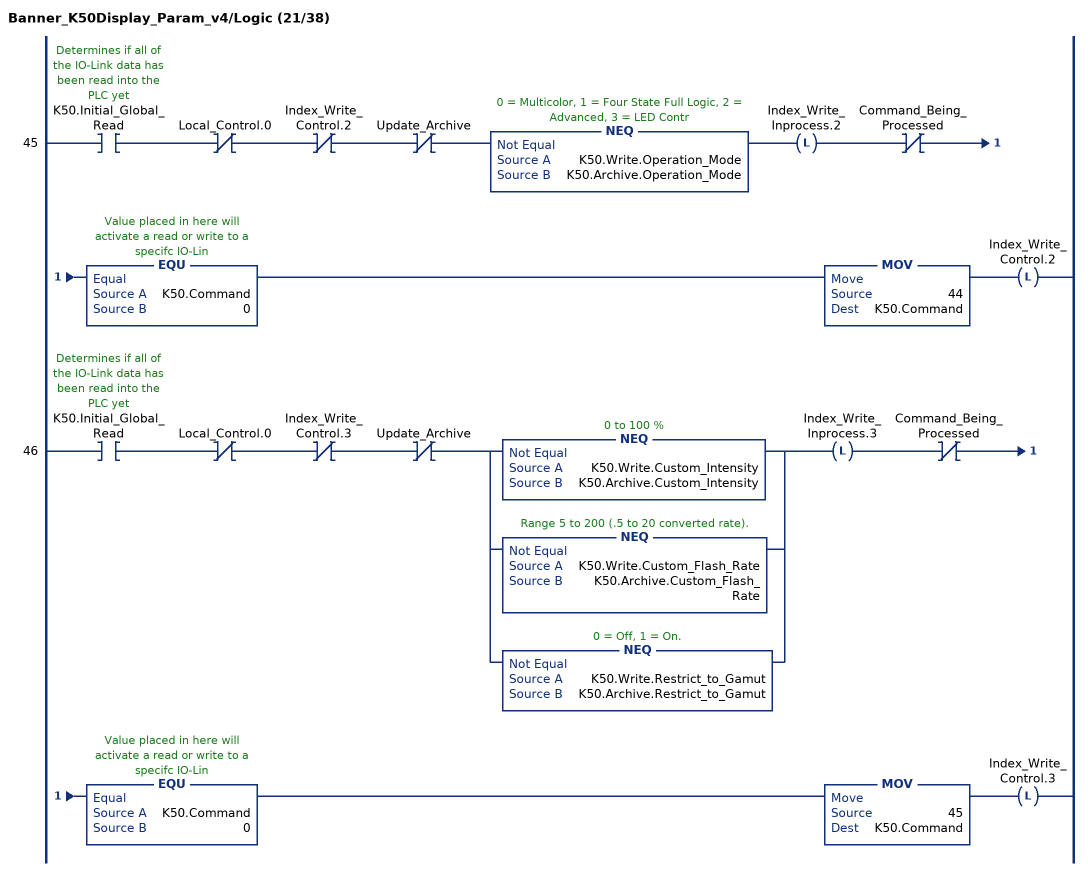
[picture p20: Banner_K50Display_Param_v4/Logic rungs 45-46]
   45: XIC(K50.Initial_Global_Read)XIO(Local_Control.0)XIO(Index_Write_Control.2)XIO(Update_Archive)NEQ(K50.Write.Operation_Mode,K50.Archive.Operation_Mode)OTL(Index_Write_Inprocess.2)XIO(Command_Being_Processed)EQU(K50.Command,0)MOV(44,K50.Command)OTL(Index_Write_Control.2);
   46: XIC(K50.Initial_Global_Read)XIO(Local_Control.0)XIO(Index_Write_Control.3)XIO(Update_Archive)[NEQ(K50.Write.Custom_Intensity,K50.Archive.Custom_Intensity) ,NEQ(K50.Write.Custom_Flash_Rate,K50.Archive.Custom_Flash_Rate) ,NEQ(K50.Write.Restrict_to_Gamut,K50.Archive.Restrict_to_Gamut) ]OTL(Index_Write_Inprocess.3)XIO(Command_Being_Processed)EQU(K50.Command,0)MOV(45,K50.Command)OTL(Index_Write_Control.3);
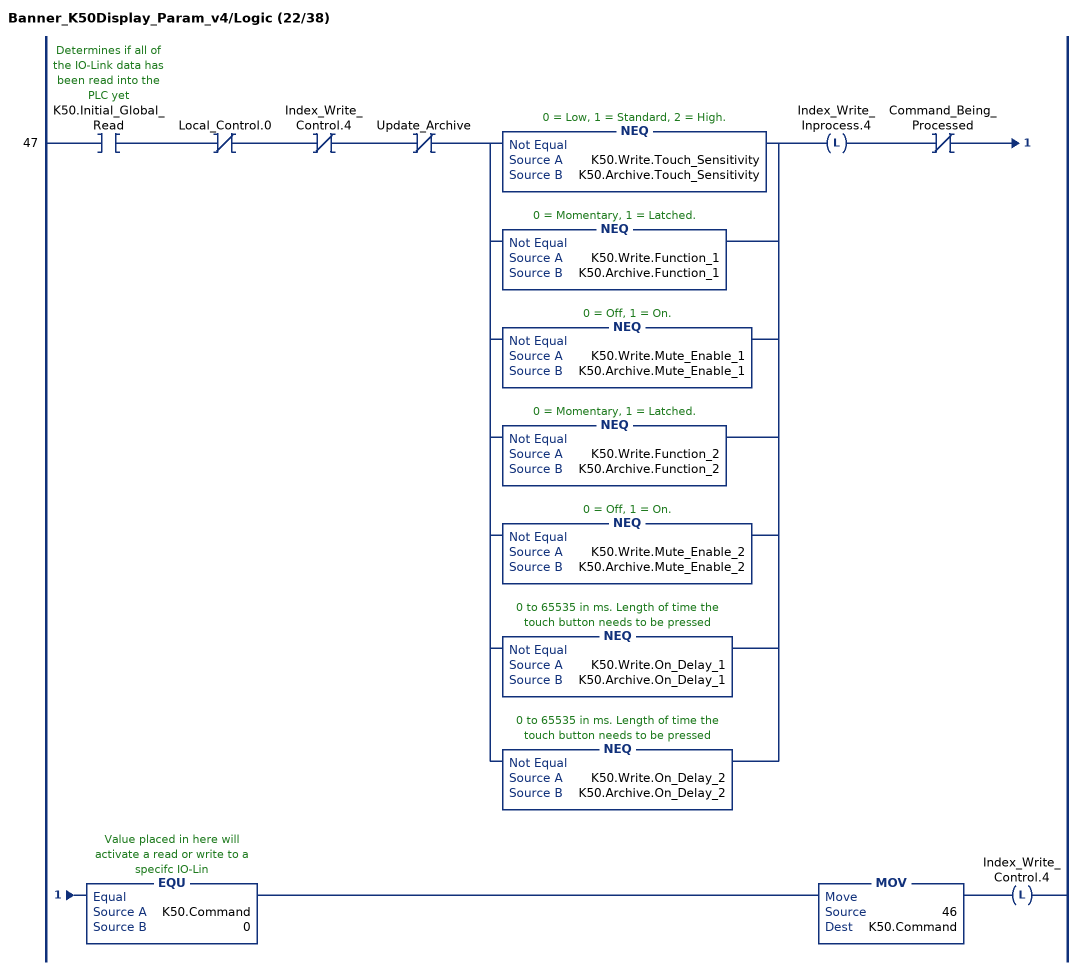
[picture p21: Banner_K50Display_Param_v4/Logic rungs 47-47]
   47: XIC(K50.Initial_Global_Read)XIO(Local_Control.0)XIO(Index_Write_Control.4)XIO(Update_Archive)[NEQ(K50.Write.Touch_Sensitivity,K50.Archive.Touch_Sensitivity) ,NEQ(K50.Write.Function_1,K50.Archive.Function_1) ,NEQ(K50.Write.Mute_Enable_1,K50.Archive.Mute_Enable_1) ,NEQ(K50.Write.Function_2,K50.Archive.Function_2) ,NEQ(K50.Write.Mute_Enable_2,K50.Archive.Mute_Enable_2) ,NEQ(K50.Write.On_Delay_1,K50.Archive.On_Delay_1) ,NEQ(K50.Write.On_Delay_2,K50.Archive.On_Delay_2) ]OTL(Index_Write_Inprocess.4)XIO(Command_Being_Processed)EQU(K50.Command,0)MOV(46,K50.Command)OTL(Index_Write_Control.4);
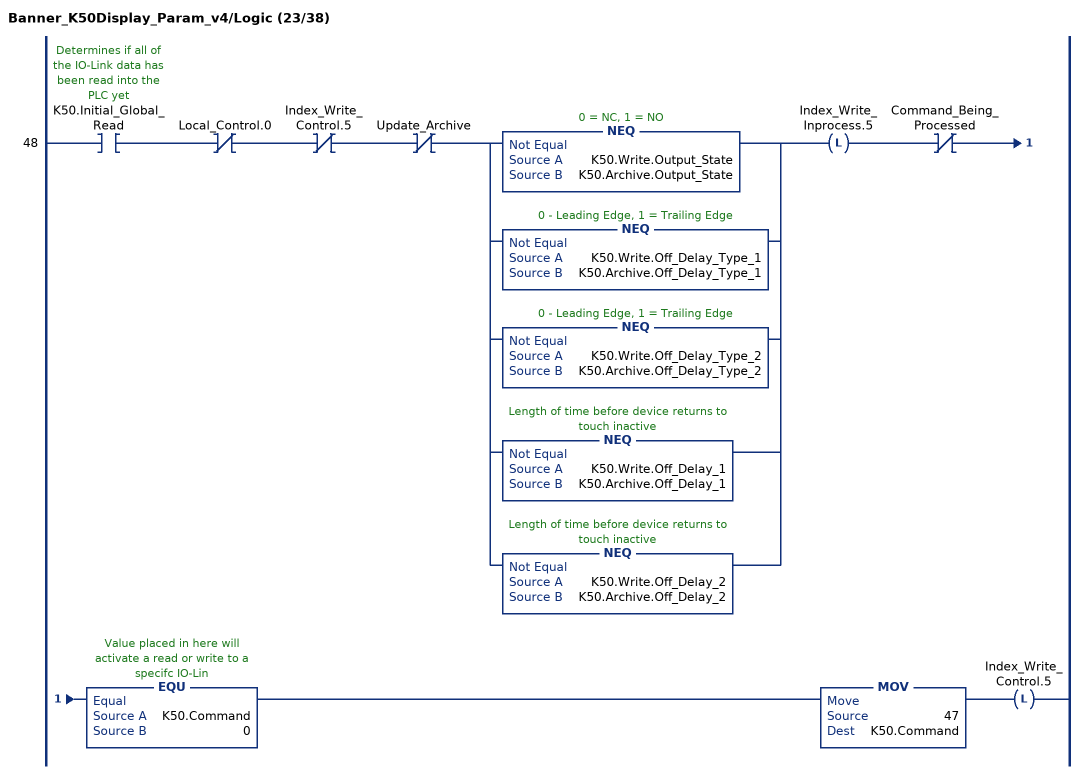
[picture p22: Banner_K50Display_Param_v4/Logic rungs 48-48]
   48: XIC(K50.Initial_Global_Read)XIO(Local_Control.0)XIO(Index_Write_Control.5)XIO(Update_Archive)[NEQ(K50.Write.Output_State,K50.Archive.Output_State) ,NEQ(K50.Write.Off_Delay_Type_1,K50.Archive.Off_Delay_Type_1) ,NEQ(K50.Write.Off_Delay_Type_2,K50.Archive.Off_Delay_Type_2) ,NEQ(K50.Write.Off_Delay_1,K50.Archive.Off_Delay_1) ,NEQ(K50.Write.Off_Delay_2,K50.Archive.Off_Delay_2) ]OTL(Index_Write_Inprocess.5)XIO(Command_Being_Processed)EQU(K50.Command,0)MOV(47,K50.Command)OTL(Index_Write_Control.5);
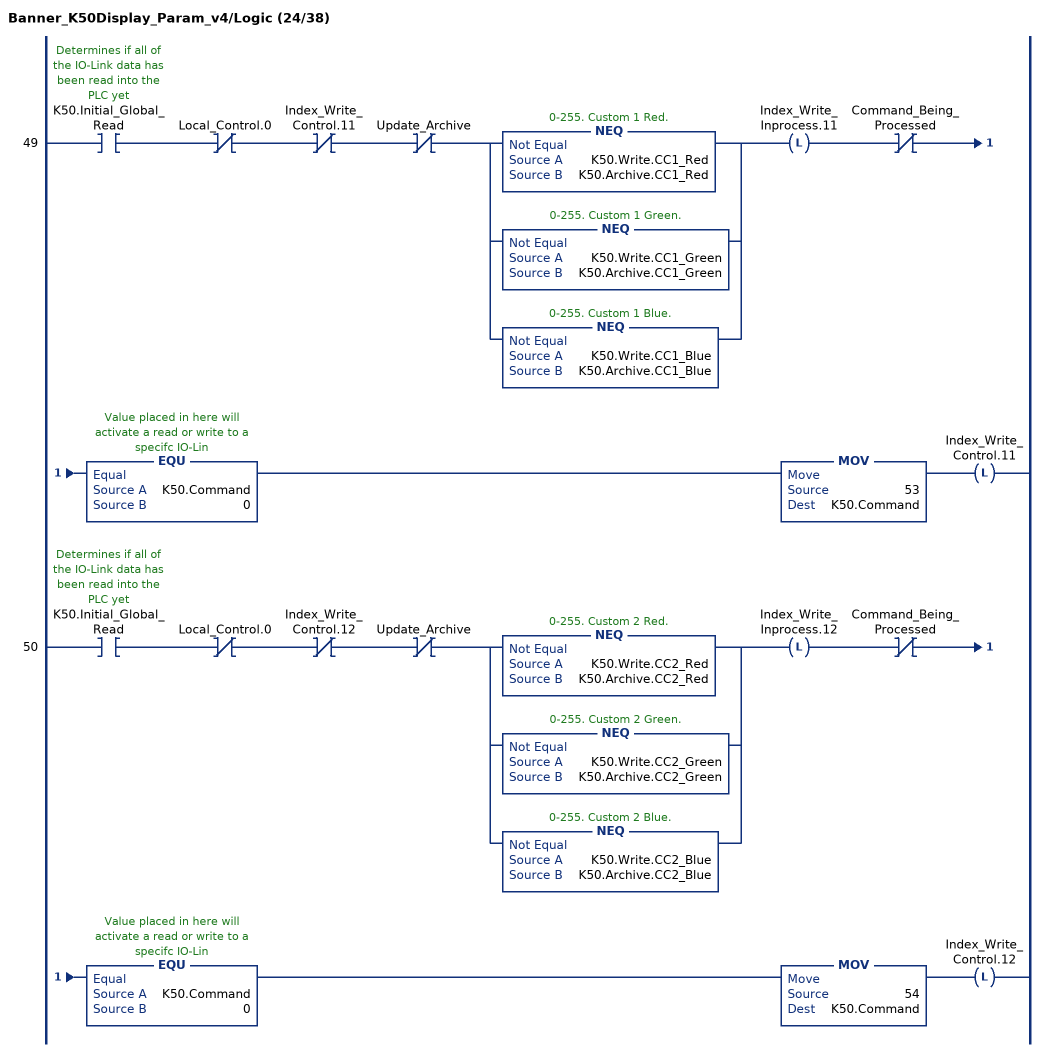
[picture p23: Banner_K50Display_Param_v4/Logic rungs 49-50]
   49: XIC(K50.Initial_Global_Read)XIO(Local_Control.0)XIO(Index_Write_Control.11)XIO(Update_Archive)[NEQ(K50.Write.CC1_Red,K50.Archive.CC1_Red) ,NEQ(K50.Write.CC1_Green,K50.Archive.CC1_Green) ,NEQ(K50.Write.CC1_Blue,K50.Archive.CC1_Blue) ]OTL(Index_Write_Inprocess.11)XIO(Command_Being_Processed)EQU(K50.Command,0)MOV(53,K50.Command)OTL(Index_Write_Control.11);
   50: XIC(K50.Initial_Global_Read)XIO(Local_Control.0)XIO(Index_Write_Control.12)XIO(Update_Archive)[NEQ(K50.Write.CC2_Red,K50.Archive.CC2_Red) ,NEQ(K50.Write.CC2_Green,K50.Archive.CC2_Green) ,NEQ(K50.Write.CC2_Blue,K50.Archive.CC2_Blue) ]OTL(Index_Write_Inprocess.12)XIO(Command_Being_Processed)EQU(K50.Command,0)MOV(54,K50.Command)OTL(Index_Write_Control.12);
